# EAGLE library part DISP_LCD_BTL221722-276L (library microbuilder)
BTL221722-276L - 2.2" 176x220 LCD Display - SPI Interface Dimensions: W: 40.3mm, L: 55mm, H: 2.35mm Logic: 1.8-3.3V VDD: 2.8-3.3V LEDs: 3*20mA LED Vf: ~3.3V
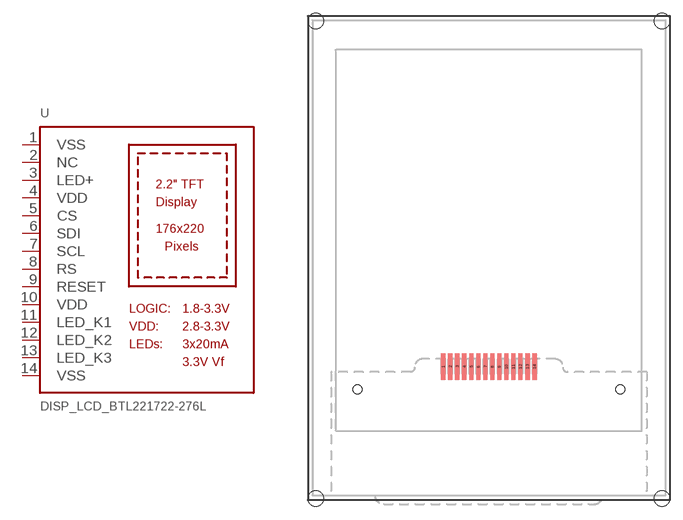
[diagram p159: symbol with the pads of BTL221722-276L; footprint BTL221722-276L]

Designator prefix U

## DISP_LCD_BTL221722-276L  [BTL221722-276L]
1  VSS  pwr
2  NC  nc
3  LED+  pwr
4  VDD  pwr
5  CS
6  SDI
7  SCL
8  RS
9  RESET
10  VDD  pwr
11  LED_K1  pwr
12  LED_K2  pwr
13  LED_K3  pwr
14  VSS  pwr

## Footprint BTL221722-276L (pad centres in mm)
smd 0.5 x 3: 1 -5.2,-16.44; 2 -4.4,-16.44; 3 -3.6,-16.44; 4 -2.8,-16.44; 5 -2,-16.44; 6 -1.2,-16.44; 7 -0.4,-16.44; 8 0.4,-16.44; 9 1.2,-16.44; 10 2,-16.44; 11 2.8,-16.44; 12 3.6,-16.44; 13 4.4,-16.44; 14 5.2,-16.44
hole 1 at -15,-19.06
hole 1 at 15,-19.06
hole 1.8 at -19.75,-31.5
hole 1.8 at 19.75,-31.5
hole 1.8 at 19.75,23
hole 1.8 at -19.75,23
